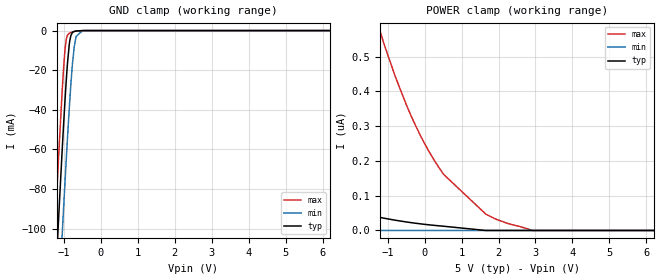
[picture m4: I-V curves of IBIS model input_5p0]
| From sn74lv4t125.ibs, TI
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|   input_5p0 Model
[Model]   input_5p0
Model_type   Input
Vinl = 0.8
Vinh = 2.02
|   typ   min   max
|   (nom PVT)   (fast PVT)   (slow PVT)
C_comp   6.617e-13   6.575e-13   6.682e-13
[Model spec]
|subparameter
Vinl   0.8   0.8   0.8
Vinh   2.02   2.02   2.1
| Where nom  PVT is Nominal Process, 5V, 40C
|   Fast PVT is Strong Process,  5.5V, -40C
|   Slow PVT is Weak Process,   4.5V, 140C
[Voltage Range]   5   4.5   5.5
|Junction Temperature
[Temperature Range]   40   140   -40
[Power Clamp Reference]   5   4.5   5.5
[GND Clamp Reference]   0   0   0
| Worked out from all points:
|   GND clamp passes 1 mA (typ) near -0.77 V on its own axis
[GND Clamp]
|   Voltage   I(typ)   I(min)   I(max)
-5V       -1.648A    -1.673A    -1.629A
-1.293V   -150.7mA   -194mA     -120mA
-1.188V   -111.4mA   -154.8mA   -80.32mA
-1.145V   -95.32mA   -138.7mA   -64.31mA
-1.044V   -59.51mA   -102.3mA   -29.66mA
-935.5mV  -24.83mA   -64.67mA   -4.359mA
-855mV    -6.918mA   -39.25mA   -1.347mA
-815mV    -2.714mA   -27.97mA   -1.014mA
-720.5mV  -422.8uA   -8.06mA    -466.3uA
-671mV    -222.5uA   -3.027mA   -270.6uA
-500mV    -17.58uA   -70.52uA   -15.37uA
10V       0A         0A         0A
[POWER Clamp]
|   Voltage   I(typ)   I(min)   I(max)
-5V       202.7nA    13.47nA    2.878uA
-3.326V   106.5nA    10.11nA    1.606uA
-3.053V   94.62nA    0A         1.437uA
-1.37V    41.17nA    0A         630.2nA
-1.14V    36.15nA    0A         550.1nA
-792.5mV  29.44nA    0A         441.9nA
-374.5mV  22.65nA    0A         331.5nA
384.5mV   13.41nA    0A         181.1nA
1.655V    0A         0A         46.98nA
2.238V    0A         0A         20.49nA
2.925V    0A         0A         0A
10V       0A         0A         0A
